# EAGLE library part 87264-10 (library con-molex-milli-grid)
RECEPTACAL
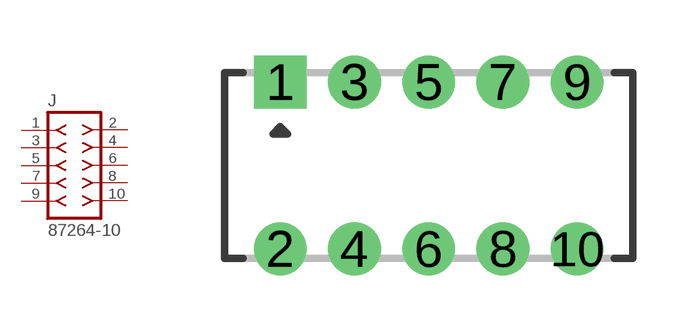
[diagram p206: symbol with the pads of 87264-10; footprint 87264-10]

Designator prefix J

## 87264-10  [87264-10]
1  1  pas
2  2  pas
3  3  pas
4  4  pas
5  5  pas
6  6  pas
7  7  pas
8  8  pas
9  9  pas
10  10  pas

## Footprint 87264-10 (pad centres in mm)
RECEPTACAL Dual Row, Side Entry
drill 0.914 square: 1 -4,2.25
drill 0.914: 2 -4,-2.25; 3 -2,2.25; 4 -2,-2.25; 5 0,2.25; 6 0,-2.25; 7 2,2.25; 8 2,-2.25; 9 4,2.25; 10 4,-2.25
